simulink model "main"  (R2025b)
settings: Solver=FixedStepAuto  StartTime=0.0  StopTime=inf  FixedStep=0.1  RelTol=1e-3
undefined symbols (not defined in the file): DiscIntNeverNeededParam
libraries: simulink_extras x2, arduinolib x1, simulink x1

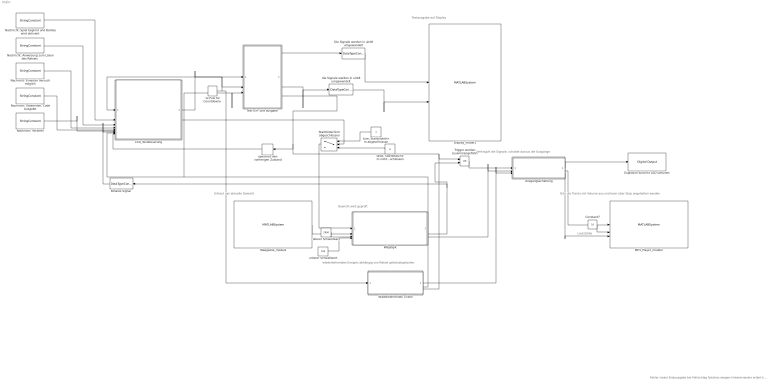
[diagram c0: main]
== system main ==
  note: Gewicht wird geprüft
  note: Lautstärke
  note: wiederkehrendes Ereignis abhängig von Rätsel gelöst/abgelaufen
  note: Verknüpft die Signale, schaltet daraus die Ausgänge
  note: Gibt die Tracks mit Volume aus und kann über Stop angehalten werden
  note: Erfasst das aktuelle Gewicht
  note: Textausgabe auf Display
  note: Fehler: keine Endausgabe bei Fehlschlag falsches wiegen hintereinander ertönt kein boom
  "1s Puls für Countdowns " : DiscretePulseGenerator  PulseType=Time based  Period=0.2  PulseWidth=50
  Ausgangsschaltung : Subsystem
  "Binäres Signal " : DataTypeConversion  OutDataTypeStr=boolean
  Constant7 : Constant  Value=10  OutDataTypeStr=uint8
  Die Signale werden in uint8 umgewandelt : DataTypeConversion  OutDataTypeStr=uint8
  Display_model1 : MATLABSystem  System=Display  SampleTime=0.1
  "Explosion wird mit LED simuliert " : arduinolib/Digital Output  pinNumber=18  Direction=output  blockPlatform=arduino
  LCD_Textsteuerung : Subsystem
  MP3_Player_model2 : MATLABSystem  System=MP3_Player  SampleTime=0.2
  "Nachricht: Anweisung zum Lösen des Rätsels " : StringConstant  String="\" Mit exakt 200ml  entschaerfst du mich!  V1=150ml, V2=250ml\""
  Nachricht: Erneuter Versuch möglich : StringConstant  String="\"Schade, aber du kannst es noch einmal versuchen !\""
  "Nachricht: Gewonnen, Code Ausgabe" : StringConstant  String="\"Herzlichen Glueckwunsch, dein Code ist        1337 !\""
  Nachricht: Spiel beginnt und Bombe wird aktiviert : StringConstant  String="\"Hallo, ich bin eine Bombe. Du hast mich gerade aktiviert !\""
  Nachricht: Verloren : StringConstant  String="\"Die Zeit hat leider nicht gereicht. Klappe den Deckel zu\""
  Startbildschirm abgeschlossen : Switch  Criteria=u2 > Threshold  Threshold=10
  Text Ein- und ausgabe : MATLAB Function  TreatAsAtomicUnit=on
  Trigger werden zusammengeführt : Logic  Operator=OR  AllPortsSameDT=off  OutDataTypeStr=boolean
  Waegzelle_model1 : MATLABSystem  System=Waegzelle  SampleTime=0.5
  Wiederkehrendes Ticken : Subsystem
  Wäglogik : Subsystem
  die Signale werden in uint8 umgewandelt : DataTypeConversion  OutDataTypeStr=uint8
  "false, Startbildschirm nicht abgeschlossen" : Constant  Value=0
  oberer Schwellwert : Constant  Value=2000
  speichert den vorherigen Zustand : Delay  DelayLength=1
  "ture, Startbildschirm abgeschlossen" : Constant
  unterer Schwellwert : Constant  Value=100
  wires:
  Constant7/1 -> MP3_Player_model2/2
  die Signale werden in uint8 umgewandelt/1 -> Display_model1/2
  Text Ein- und ausgabe/2(row_idx) -> die Signale werden in uint8 umgewandelt/1
  Die Signale werden in uint8 umgewandelt/1 -> Display_model1/1
  Text Ein- und ausgabe/1(text_line) -> Die Signale werden in uint8 umgewandelt/1
  "1s Puls für Countdowns "/1 -> Wiederkehrendes Ticken/1(Puls), LCD_Textsteuerung/1(In Puls), Text Ein- und ausgabe/2(pulse_trigger)
  "false, Startbildschirm nicht abgeschlossen"/1 -> Startbildschirm abgeschlossen/3
  "ture, Startbildschirm abgeschlossen"/1 -> Startbildschirm abgeschlossen/1
  Text Ein- und ausgabe/4(timer_done) -> Wiederkehrendes Ticken/3(Rätsel abgelaufen), Trigger werden zusammengeführt/1, speichert den vorherigen Zustand/1
  Wäglogik/1(Wagge korrektes Gewicht) -> Wiederkehrendes Ticken/2(Rätsel gelöst), Text Ein- und ausgabe/3(stop_signal), LCD_Textsteuerung/8(In Stop bei Erfolg)
  Wäglogik/2(Waage falsches Gewicht) -> "Binäres Signal "/1, Trigger werden zusammengeführt/2
  Startbildschirm abgeschlossen/1 -> Wäglogik/1(Eingang Wägprozess starten)
  Waegzelle_model1/1 -> Wäglogik/2(Eingang Gewicht)
  oberer Schwellwert/1 -> Wäglogik/3(In oberer Schwellwert)
  unterer Schwellwert/1 -> Wäglogik/4(In unterer Schwellwert)
  Nachricht: Spiel beginnt und Bombe wird aktiviert/1 -> LCD_Textsteuerung/2(Begrüßungstext)
  "Nachricht: Anweisung zum Lösen des Rätsels "/1 -> LCD_Textsteuerung/3(Anweisungstext)
  Nachricht: Erneuter Versuch möglich/1 -> LCD_Textsteuerung/4(Failtext)
  "Nachricht: Gewonnen, Code Ausgabe"/1 -> LCD_Textsteuerung/5(Erfolgstext)
  Nachricht: Verloren/1 -> LCD_Textsteuerung/6(Komplett Versagt)
  speichert den vorherigen Zustand/1 -> LCD_Textsteuerung/9(In Zeit abgelaufen)
  "Binäres Signal "/1 -> LCD_Textsteuerung/7(In Waage falsches Gewicht)
  LCD_Textsteuerung/1(Out Display) -> Text Ein- und ausgabe/1(full_text)
  LCD_Textsteuerung/2(Out Startausgabe abgeschlossen) -> Startbildschirm abgeschlossen/2
  Ausgangsschaltung/2(Out MP3 Track1) -> MP3_Player_model2/1
  Ausgangsschaltung/1(Out LED Streifen1) -> "Explosion wird mit LED simuliert "/1
  Ausgangsschaltung/3(Out MP3 Stop1) -> MP3_Player_model2/3
  Wäglogik/3(MP3_Ausgang unlocked) -> Ausgangsschaltung/2(In Track unlocked1)
  Wiederkehrendes Ticken/1(Spiele Track 3) -> Ausgangsschaltung/3(In Track Uhr1)
  Trigger werden zusammengeführt/1 -> Ausgangsschaltung/1(In Track Explosion1)

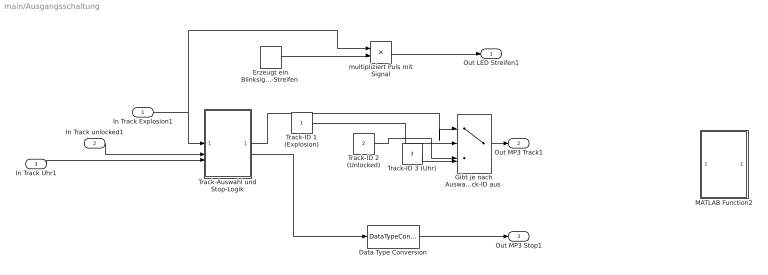
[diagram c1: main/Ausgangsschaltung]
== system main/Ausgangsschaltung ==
  In Track Explosion1 : Inport
  In Track unlocked1 : Inport  Port=2
  In Track Uhr1 : Inport  Port=3
  Data Type Conversion : DataTypeConversion  OutDataTypeStr=boolean
  "Erzeugt ein Blinksignal für den LED-Streifen " : DiscretePulseGenerator  PulseType=Time based  Period=1  PulseWidth=50
  "Gibt je nach Auswahl die passende Track-ID aus " : MultiPortSwitch  Inputs=4
  MATLAB Function2 : MATLAB Function  Commented=on  TreatAsAtomicUnit=on
  Track-Auswahl und Stop-Logik : MATLAB Function  TreatAsAtomicUnit=on
  Track-ID 1 (Explosion) : Constant  OutDataTypeStr=uint8
  Track-ID 2 (Unlocked) : Constant  Value=2  OutDataTypeStr=uint8
  Track-ID 3 (Uhr) : Constant  Value=3  OutDataTypeStr=uint8
  multipliziert Puls mit Signal : Product
  Out LED Streifen1 : Outport
  Out MP3 Track1 : Outport  Port=2
  Out MP3 Stop1 : Outport  Port=3
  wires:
  Track-ID 1 (Explosion)/1 -> "Gibt je nach Auswahl die passende Track-ID aus "/2
  Track-ID 2 (Unlocked)/1 -> "Gibt je nach Auswahl die passende Track-ID aus "/3
  Track-ID 3 (Uhr)/1 -> "Gibt je nach Auswahl die passende Track-ID aus "/4
  In Track unlocked1/1 -> Track-Auswahl und Stop-Logik/2(u2)
  In Track Uhr1/1 -> Track-Auswahl und Stop-Logik/3(u3)
  "Gibt je nach Auswahl die passende Track-ID aus "/1 -> Out MP3 Track1/1
  In Track Explosion1/1 -> multipliziert Puls mit Signal/1, Track-Auswahl und Stop-Logik/1(u1)
  multipliziert Puls mit Signal/1 -> Out LED Streifen1/1
  "Erzeugt ein Blinksignal für den LED-Streifen "/1 -> multipliziert Puls mit Signal/2
  Track-Auswahl und Stop-Logik/1(y) -> "Gibt je nach Auswahl die passende Track-ID aus "/1
  Track-Auswahl und Stop-Logik/2(stop) -> Data Type Conversion/1
  Data Type Conversion/1 -> Out MP3 Stop1/1

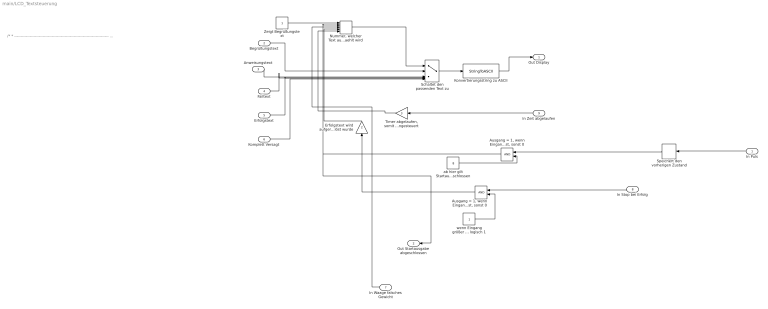
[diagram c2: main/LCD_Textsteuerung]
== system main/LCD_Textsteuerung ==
  note: /* * ------------------------------------------------------------------------- * Funktion: hx711_init_sensor * ------------------------------------------------------------------------- * Beschreibung: Initialisiert den HX711 (Pinbelegung) und setzt den * Kalibrierungsfaktor. Führt beim Start eine Tara (Nullabgleich) durch, * sodass die aktuelle Last als "0" behandelt wird. * * Hinweis: Der Kalibrierungsfaktor muss vorher ermittelt werden. * Wird 0.0 übergeben, wird 1.0 als Default gesetzt, damit * eine gültige Skalierung vorhanden ist (nahe an Rohwerten). * * Eingänge: * - dout: Data-Out Pin (DOUT) des HX711 * - sck: Clock Pin (SCK) des HX711 * - scale_factor: Kalibrierungsfaktor (Rohwert -> Gewichtseinheit) * * Ausgänge: Keine * Ersteller: Tobias Brandt, Seda Ünal * Datum: 20.11.2025 * Letzte Änderung: 14.12.2025 * ------------------------------------------------------------------------- */
  In Puls : Inport
  Begrüßungstext : Inport  Port=2
  Anweisungstext : Inport  Port=3
  Failtext : Inport  Port=4
  Erfolgstext : Inport  Port=5
  Komplett Versagt : Inport  Port=6
  In Waage falsches Gewicht : Inport  Port=7
  In Stop bei Erfolg : Inport  Port=8
  In Zeit abgelaufen : Inport  Port=9
  "Ausgang = 1, wenn Eingang größer/gleich dem Schwellwert ist, sonst 0" : RelationalOperator  OutDataTypeStr=boolean  RndMeth=Simplest
  "Ausgang = 1, wenn Eingang mindestens 1 ist, sonst 0" : RelationalOperator  OutDataTypeStr=boolean  RndMeth=Simplest
  "Erfolgstext wird aufgerufen, wenn Spiel erfolgreich gelöst wurde" : Gain  Gain=2
  Konvertierungsstring zu ASCII : StringToASCII  OutputVectorSize=82
  "Nummer, welcher Text ausgewaehlt wird" : Sum  Inputs=+++++
  Schaltet den passenden Text zu : MultiPortSwitch  Inputs=5
  Speichert den vorherigen Zustand : DiscreteIntegrator  SampleTime=-1  ICPrevOutput=DiscIntNeverNeededParam  ICPrevScaledInput=DiscIntNeverNeededParam
  "Timer abgelaufen, somit wird komplett versagt Text angesteuert" : Gain  Gain=3
  Zeigt Begrüßungstext : Constant
  ab hier gilt Startausgabe als abgeschlossen : Constant  Value=8
  "wenn Eingang größer 1, Ausgang logisch 1" : Constant
  Out Display : Outport
  Out Startausgabe abgeschlossen : Outport  Port=2
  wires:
  In Zeit abgelaufen/1 -> "Timer abgelaufen, somit wird komplett versagt Text angesteuert"/1
  "wenn Eingang größer 1, Ausgang logisch 1"/1 -> "Ausgang = 1, wenn Eingang mindestens 1 ist, sonst 0"/2
  "Nummer, welcher Text ausgewaehlt wird"/1 -> Schaltet den passenden Text zu/1
  "Ausgang = 1, wenn Eingang größer/gleich dem Schwellwert ist, sonst 0"/1 -> "Nummer, welcher Text ausgewaehlt wird"/2, Out Startausgabe abgeschlossen/1
  "Timer abgelaufen, somit wird komplett versagt Text angesteuert"/1 -> "Nummer, welcher Text ausgewaehlt wird"/5
  Schaltet den passenden Text zu/1 -> Konvertierungsstring zu ASCII/1
  ab hier gilt Startausgabe als abgeschlossen/1 -> "Ausgang = 1, wenn Eingang größer/gleich dem Schwellwert ist, sonst 0"/2
  In Waage falsches Gewicht/1 -> "Nummer, welcher Text ausgewaehlt wird"/3
  Speichert den vorherigen Zustand/1 -> "Ausgang = 1, wenn Eingang größer/gleich dem Schwellwert ist, sonst 0"/1
  "Ausgang = 1, wenn Eingang mindestens 1 ist, sonst 0"/1 -> "Erfolgstext wird aufgerufen, wenn Spiel erfolgreich gelöst wurde"/1
  Zeigt Begrüßungstext/1 -> "Nummer, welcher Text ausgewaehlt wird"/1
  "Erfolgstext wird aufgerufen, wenn Spiel erfolgreich gelöst wurde"/1 -> "Nummer, welcher Text ausgewaehlt wird"/4
  Erfolgstext/1 -> Schaltet den passenden Text zu/5
  Anweisungstext/1 -> Schaltet den passenden Text zu/3
  Konvertierungsstring zu ASCII/1 -> Out Display/1
  Begrüßungstext/1 -> Schaltet den passenden Text zu/2
  In Stop bei Erfolg/1 -> "Ausgang = 1, wenn Eingang mindestens 1 ist, sonst 0"/1
  Failtext/1 -> Schaltet den passenden Text zu/4
  Komplett Versagt/1 -> Schaltet den passenden Text zu/6
  In Puls/1 -> Speichert den vorherigen Zustand/1

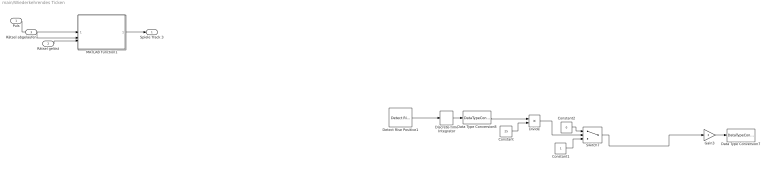
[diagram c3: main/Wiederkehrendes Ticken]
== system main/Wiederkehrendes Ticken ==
  Puls : Inport
  Rätsel gelöst : Inport  Port=2
  Rätsel abgelaufen : Inport  Port=3
  Constant : Constant  Commented=on  Value=25
  Constant1 : Constant  Commented=on
  Constant2 : Constant  Commented=on  Value=0
  Data Type Conversion7 : DataTypeConversion  Commented=on  OutDataTypeStr=uint8
  Data Type Conversion8 : DataTypeConversion  Commented=on  OutDataTypeStr=uint8
  Detect Rise Positive1 : simulink/Logic and Bit Operations/Detect Rise Positive  Commented=on  vinit=0  OutDataTypeStr=boolean
  Discrete-Time Integrator : DiscreteIntegrator  Commented=on  SampleTime=-1  ICPrevOutput=DiscIntNeverNeededParam  ICPrevScaledInput=DiscIntNeverNeededParam
  Divide : Product  Commented=on  Inputs=*/
  Gain3 : Gain  Commented=on  Gain=3
  MATLAB Function1 : MATLAB Function  TreatAsAtomicUnit=on
  Switch7 : Switch  Commented=on  Threshold=1
  Spiele Track 3 : Outport
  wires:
  MATLAB Function1/1(trigger_out) -> Spiele Track 3/1
  Divide/1 -> Switch7/2
  Discrete-Time Integrator/1 -> Data Type Conversion8/1
  Data Type Conversion8/1 -> Divide/1
  Constant2/1 -> Switch7/1
  Switch7/1 -> Gain3/1
  Constant/1 -> Divide/2
  Detect Rise Positive1/1 -> Discrete-Time Integrator/1
  ? -> Detect Rise Positive1/1
  Constant1/1 -> Switch7/3
  Gain3/1 -> Data Type Conversion7/1
  Puls/1 -> MATLAB Function1/1(clk_puls)
  Rätsel gelöst/1 -> MATLAB Function1/3(puz_solve)
  Rätsel abgelaufen/1 -> MATLAB Function1/2(puz_fail)

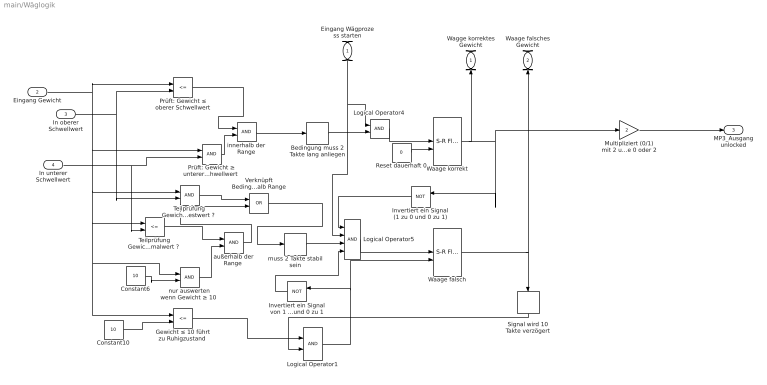
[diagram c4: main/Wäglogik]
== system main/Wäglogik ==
  Eingang Wägprozess starten : Inport
  Eingang Gewicht : Inport  Port=2
  In oberer Schwellwert : Inport  Port=3
  In unterer Schwellwert : Inport  Port=4
  Bedingung muss 2 Takte lang anliegen : Delay
  Constant10 : Constant  Value=10
  Constant6 : Constant  Value=10
  "Gewicht ≤ 10 führt zu Ruhigzustand " : RelationalOperator  Operator=<=  OutDataTypeStr=boolean  RndMeth=Simplest
  Invertiert ein Signal (1 zu 0 und 0 zu 1) : Logic  Operator=NOT  IconShape=distinctive  AllPortsSameDT=off  OutDataTypeStr=boolean
  Invertiert ein Signal von 1 zu 0 und 0 zu 1 : Logic  Operator=NOT  IconShape=distinctive  AllPortsSameDT=off  OutDataTypeStr=boolean
  Logical Operator1 : Logic  AllPortsSameDT=off  OutDataTypeStr=boolean
  Logical Operator4 : Logic  AllPortsSameDT=off  OutDataTypeStr=boolean
  Logical Operator5 : Logic  Inputs=4  AllPortsSameDT=off  OutDataTypeStr=boolean
  Multipliziert (0/1) mit 2 und erzeugt Code 0 oder 2 : Gain  Gain=2
  Prüft: Gewicht ≤ oberer Schwellwert : RelationalOperator  Operator=<=  OutDataTypeStr=boolean  RndMeth=Simplest
  "Prüft: Gewicht ≥ unterer Schwellwert " : RelationalOperator  OutDataTypeStr=boolean  RndMeth=Simplest
  Reset dauerhaft 0 : Constant  Value=0  OutDataTypeStr=boolean
  Signal wird 10 Takte verzögert : Delay  DelayLength=10
  "Teilprüfung Gewicht unter Maximalwert ? " : RelationalOperator  Operator=<=  OutDataTypeStr=boolean  RndMeth=Simplest
  "Teilprüfung Gewicht über Mindestwert ? " : RelationalOperator  OutDataTypeStr=boolean  RndMeth=Simplest
  Verknüpft Bedingungen für außerhalb Range : Logic  Operator=OR  IconShape=distinctive  AllPortsSameDT=off  OutDataTypeStr=boolean
  Waage falsch : simulink_extras/Flip Flops/S-R Flip-Flop  initial_condition=0
  Waage korrekt : simulink_extras/Flip Flops/S-R Flip-Flop  initial_condition=0
  "außerhalb der Range " : Logic  AllPortsSameDT=off  OutDataTypeStr=boolean
  innerhalb der Range : Logic  AllPortsSameDT=off  OutDataTypeStr=boolean
  muss 2 Takte stabil sein : Delay
  "nur auswerten wenn Gewicht ≥ 10 " : RelationalOperator  OutDataTypeStr=boolean  RndMeth=Simplest
  Wagge korrektes Gewicht : Outport
  Waage falsches Gewicht : Outport  Port=2
  MP3_Ausgang unlocked : Outport  Port=3
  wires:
  Bedingung muss 2 Takte lang anliegen/1 -> Logical Operator4/2
  muss 2 Takte stabil sein/1 -> Logical Operator5/3
  Waage falsch/1 -> Waage falsches Gewicht/1, Signal wird 10 Takte verzögert/1
  "nur auswerten wenn Gewicht ≥ 10 "/1 -> "außerhalb der Range "/2
  Logical Operator1/1 -> Waage falsch/2, Invertiert ein Signal von 1 zu 0 und 0 zu 1/1
  Invertiert ein Signal von 1 zu 0 und 0 zu 1/1 -> Logical Operator5/4
  In unterer Schwellwert/1 -> "Prüft: Gewicht ≥ unterer Schwellwert "/2, "Teilprüfung Gewicht unter Maximalwert ? "/2
  innerhalb der Range/1 -> Bedingung muss 2 Takte lang anliegen/1
  In oberer Schwellwert/1 -> "Teilprüfung Gewicht über Mindestwert ? "/2, Prüft: Gewicht ≤ oberer Schwellwert/2
  Eingang Wägprozess starten/1 -> Logical Operator4/1, Logical Operator5/2
  Constant10/1 -> "Gewicht ≤ 10 führt zu Ruhigzustand "/2
  Invertiert ein Signal (1 zu 0 und 0 zu 1)/1 -> Logical Operator5/1
  "Gewicht ≤ 10 führt zu Ruhigzustand "/1 -> Logical Operator1/1
  "außerhalb der Range "/1 -> Verknüpft Bedingungen für außerhalb Range/2
  Constant6/1 -> "nur auswerten wenn Gewicht ≥ 10 "/2
  Verknüpft Bedingungen für außerhalb Range/1 -> muss 2 Takte stabil sein/1
  "Teilprüfung Gewicht über Mindestwert ? "/1 -> Verknüpft Bedingungen für außerhalb Range/1
  Logical Operator5/1 -> Waage falsch/1
  Signal wird 10 Takte verzögert/1 -> Logical Operator1/2
  Eingang Gewicht/1 -> Prüft: Gewicht ≤ oberer Schwellwert/1, "Gewicht ≤ 10 führt zu Ruhigzustand "/1, "nur auswerten wenn Gewicht ≥ 10 "/1, "Teilprüfung Gewicht unter Maximalwert ? "/1, "Teilprüfung Gewicht über Mindestwert ? "/1, "Prüft: Gewicht ≥ unterer Schwellwert "/1
  "Teilprüfung Gewicht unter Maximalwert ? "/1 -> "außerhalb der Range "/1
  Reset dauerhaft 0/1 -> Waage korrekt/2
  Prüft: Gewicht ≤ oberer Schwellwert/1 -> innerhalb der Range/1
  Waage korrekt/1 -> Multipliziert (0/1) mit 2 und erzeugt Code 0 oder 2/1, Invertiert ein Signal (1 zu 0 und 0 zu 1)/1, Wagge korrektes Gewicht/1
  "Prüft: Gewicht ≥ unterer Schwellwert "/1 -> innerhalb der Range/2
  Logical Operator4/1 -> Waage korrekt/1
  Multipliziert (0/1) mit 2 und erzeugt Code 0 oder 2/1 -> MP3_Ausgang unlocked/1

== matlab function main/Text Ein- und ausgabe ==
function [text_line, row_idx, write_enable, timer_done] = typewriter_output(full_text, pulse_trigger, stop_signal)
%#codegen
persistent cursor timer_sec active_timer text_done tick_counter timer_finished_mem display_cycle;   % Zustände bleiben zwischen Aufrufen erhalten
if isempty(cursor)                                                                                  % Initialisierung nur beim ersten Aufruf
    cursor = int32(1);                                                                              % Aktueller „Tipppunkt“ (1-basiert)
    timer_sec = int32(300);                                                                         % Countdown in 300ms
    active_timer = false;                                                                           % Timer läuft erst nach kompletter Textausgabe
    text_done = false;                                                                              % Text ist am Anfang noch nicht vollständig
    tick_counter = int32(0);                                                                        % Zähler für Ticks
    timer_finished_mem = false;                                                                     % Timer ist noch nicht abgelaufen
    display_cycle = int32(0);                                                                       % Platzhalter für Anzeige-Zyklus
end
len_text = int32(numel(full_text));                                                                 % Textlänge als int32

if pulse_trigger                                                                                    % Zustand wird nur bei Impul weitgerfüjrt 
    % A) --Schreibmaschine (Initialer Textaufbau)--
    if ~text_done                                                                                   
        if cursor < len_text
            cursor = cursor + 1;                                                                    % Ein weiteres Zeichen sichtbar machen
        else
            text_done = true;                                                                       % Text ist vollständig
            active_timer = true;                                                                    % Timer ist aktiv
            tick_counter = int32(0);                                                                % Rotation wird sauber gestartet
        end
    end
    
    % B) --Timer Countdown & Anzeige-Zyklus Logik--
    if text_done
      
       
        tick_counter = tick_counter + 1;                                                            % Der Tick wird IMMER hochgezählt, damit der Text rotiert
        
        
        if tick_counter >= 5                                                                        % 5 Ticks Zyklus
            
           
            if active_timer                                                                         % Timer Logik: Nur hier prüfen wir das Stop-Signal
                if timer_sec > 0
                    if stop_signal == 0                                                             % Nur herunterzählen, wenn kein Stop-Signal anliegt

                        timer_sec = timer_sec - int32(1);
                    end
                else
                    timer_finished_mem = true;
                    active_timer = false;
                end
            end
            
            
            tick_counter = int32(0);                                                                % Reset muss immer passieren, damit die Anzeige rotiert
        end
    end
end

timer_done = uint8(timer_finished_mem);

                                                                                                     %% --2. Ausgabe-Logik--
text_line = uint8(32 * ones(20, 1));
if ~text_done
                                                                                                     %% --Modus A: Schreibmaschine--
    current_row_dbl = floor(double(cursor - 1) / 20);                                               
    row_idx = uint8(current_row_dbl);
    start_of_row = int32(current_row_dbl * 20 + 1);
    chars_in_this_row = cursor - (start_of_row - 1);                                                 % sichtbare Zeichen in dieser Zeile
    if chars_in_this_row > 20;
        chars_in_this_row = int32(20);                                                               % LCD hat nur 20 Spalten
    end
    
    if chars_in_this_row > 0
        for k = 1:chars_in_this_row
            char_pos = start_of_row + k - 1;
            if char_pos <= len_text
                text_line(k) = uint8(full_text(char_pos));                                           % ASCII-Code übernehmen
            end
        end
    end
else
                                                                                                     %% --Modus B: Synchronisierter Timer--
    
                                                                                                     % Tick 0 -> Zeile 0
                                                                                                     % Tick 1 -> Zeile 1
                                                                                                     % Tick 2 -> Zeile 2
                                                                                                     % Tick 3 & 4 -> Zeile 3 (Timer)
    
    if tick_counter <= 2
        current_show_row = tick_counter;
    else
        current_show_row = int32(3);
    end
    
    row_idx = uint8(current_show_row);
    
    if current_show_row < 3
                                                                                                     % --Statischer Text--
        start_idx = int32(current_show_row * 20 + 1);                                                % Startindex des Textblocks
        for k = 1:20
            idx = start_idx + k - 1;                                                                 % Index im full_text
            if idx <= len_text
                text_line(k) = uint8(full_text(idx));
            else
                text_line(k) = uint8(32); 
            end
        end
    else
                                                                                                     % --Timer anzeigen--
        row_idx = uint8(3); 
        minutes = int32(floor(double(timer_sec) / 60));
        seconds = int32(mod(double(timer_sec), 60));
        
        timer_str = uint8(32 * ones(5, 1));
        timer_str(1) = uint8('0') + uint8(floor(double(minutes)/10));
        timer_str(2) = uint8('0') + uint8(mod(double(minutes),10));
        timer_str(3) = uint8(':');
        timer_str(4) = uint8('0') + uint8(floor(double(seconds)/10));
        timer_str(5) = uint8('0') + uint8(mod(double(seconds),10));
        
        text_line(8:12) = timer_str;                                                                 % Timer mittig platzieren (Spalten 8:12)
    end
end
write_enable = uint8(1);                                                                             % Display darf aktualisiert werden
end

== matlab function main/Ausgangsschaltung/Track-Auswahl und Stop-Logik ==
function [y, stop] = fcn(u1, u2, u3)
                                                                  %% 1. --Eingangskonvertierung--
    u1_d = double(u1);
    u2_d = double(u2);
    u3_d = double(u3);
    
                                                                  %% 2. --Zustände merken--
                                                                  % timer_active: Zählt runter, wie lange ein Track noch anliegen soll
                                                                  % active_track: Merkt sich, welcher Track gerade spielt
    persistent u1_alt u2_alt timer_active active_track
    
    if isempty(u1_alt)
        u1_alt = 0; u2_alt = 0;
        timer_active = 0;
        active_track = 0;
    end
    
   
    
                                                                  %% A) --Eingänge Prüfen-- (Priorität: Explosion > Lösen > Uhr)
    
                                                                  % 1.Explosion,startet nur bei 0->1 Übergang
    if (u1_d > 0) && (u1_alt <= 0)
        active_track = 1;
        timer_active = 5; % Signal für 5 Ticks (1 Sekunde) halten
    end
    
                                                                  % 2.Flankenerkennung, nur wenn Explosion nicht aktiv gestartet wurde
    if (u2_d > 0) && (u2_alt <= 0) && (active_track ~= 1)
        active_track = 2;
        timer_active = 5; % Signal für 5 Ticks (1 Sekunde) halten
    end
    
                                                                  % 3. Uhr,Pegelerkennung
                                                                  % Wenn Uhr kommt und gerade nichts Wichtigeres läuft (Timer 0)
    if (u3_d > 0) && (timer_active == 0)
        active_track = 3;
        timer_active = 1; 
    end
    
    
                                                                  %% --Ausgabe Logik--
    
    if timer_active > 0
        y = active_track;                                         % Den gespeicherten Track ausgeben
        stop = 0;                                                 % Spielen erlauben!
        
                                                                  % Timer runterzählen (außer bei Uhr, die steuert sich über Eingang u3 selbst,
                                                                  % aber kurzes Runterzählen schadet nicht für saubere Übergänge)
        timer_active = timer_active - 1; 
    else
        y = 0;
        active_track = 0;     % Reset
        stop = 1;             % Jetzt erst Stop senden
    end
    
                                                                  %% 4.--Zustand speichern--
    u1_alt = u1_d;
    u2_alt = u2_d;
end

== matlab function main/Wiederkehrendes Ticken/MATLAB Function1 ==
function trigger_out = fcn(clk_puls, puz_fail, puz_solve)
    persistent timer_count                                                                    % merkt sich den Zählerstand über mehrere Funktionsaufrufe hinweg
    
    if isempty(timer_count)
        timer_count = 0;
    end
    
    trigger_out = 0;

   
    if (puz_fail == 0) && (puz_solve == 0)                                                     % Nur ausführen, wenn Rätsel noch läuft
        
       
        if clk_puls == 1                                                                       % Eingang: Puls alle 0,2s
            timer_count = timer_count + 1;
        end
        
                                                                                               % Zustandsprüfung:
                                                                                               % 30 Sekunden = 150 Pulse (bei 0,2s Takt)
                                                                                               % 1 Sekunde   = 5 Pulse
        
                                                                                               % Schritt A: 30s sind erreicht. 
                                                                                               % Wir halten das Signal für 5 Pulse (5 * 0,2s = 1s), also bis Zähler 155 erreicht.
        
        if (timer_count >= 150) && (timer_count < 155)
            trigger_out = 3; 
            
                                                                                               % Schritt B: Nach den 5 aktiven Pulsen (bei 155) resetten wir.
        elseif timer_count >= 155
            timer_count = 0; 
            trigger_out = 0; 
            
        else
                                                                                               % Zähler ist noch beim Hochzählen (0 bis 149)
            trigger_out = 0;
        end
        
    else
                                                                                               % Reset, wenn Rätsel vorbei
        timer_count = 0;
        trigger_out = 0;
    end

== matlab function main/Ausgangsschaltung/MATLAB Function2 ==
function [y, stop] = fcn(u1, u2, u3)
    % 1. EINGANGSKONVERTIERUNG
    u1_d = double(u1);
    u2_d = double(u2);
    u3_d = double(u3);
    
    % 2. GEDÄCHTNIS (nur noch für Flankenerkennung von u1/u2 nötig)
    persistent u1_alt u2_alt
    if isempty(u1_alt)
        u1_alt = 0; u2_alt = 0; 
    end
    
    % Standardwert: Nichts abspielen
    y = 0;      
    
    % --- LOGIK ---
    % Wir prüfen die Eingänge nacheinander. Da wir kein "elseif" verwenden, 
    % blockieren alte Zustände (wie "Spiel vorbei") nicht die neuen Signale.
    % Der jeweils letzte aktive Befehl im Code gewinnt für den aktuellen Zeitschritt.

    % A) UHR (Track 3)
    % Da das Signal u3 für 1s anliegt, geben wir solange 3 aus.
    if u3_d > 0
        y = 3;
    end
    
    % B) RÄTSEL GELÖST (Track 2)
    % Reagiert nur auf die steigende Flanke (0 -> 1)
    if (u2_d > 0) && (u2_alt <= 0)
        y = 2; 
    end
        
    % C) EXPLOSION (Track 1)
    % Reagiert nur auf die steigende Flanke (0 -> 1)
    if (u1_d > 0) && (u1_alt <= 0)
        y = 1; 
    end
    
    
    % --- STOP LOGIK ---
    % Wenn ein Track ausgewählt ist (y > 0), muss Stop auf 0 (Play) gehen.
    % Wenn y == 0 ist, senden wir Stop = 1.
    if y > 0
        stop = 0;
    else
        stop = 1;
    end
    
    % 4. ZUSTAND SPEICHERN
    u1_alt = u1_d;
    u2_alt = u2_d;
end
